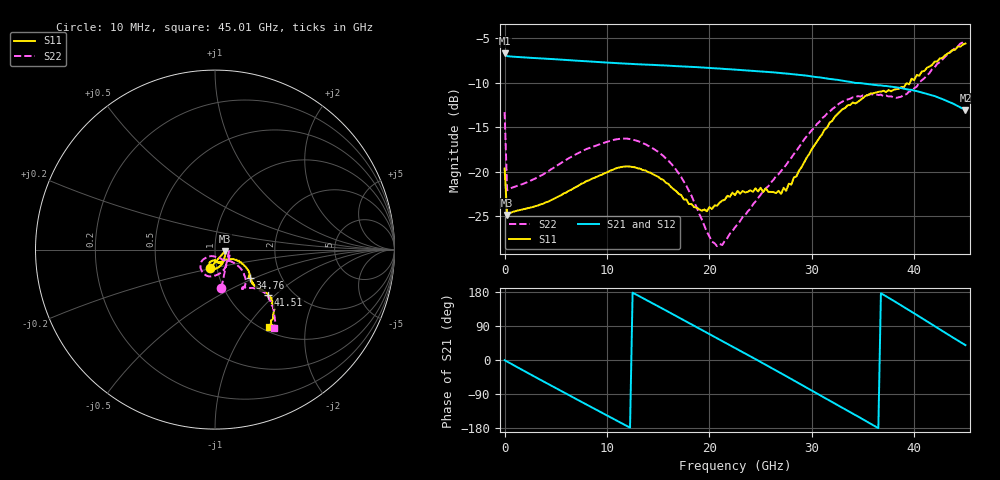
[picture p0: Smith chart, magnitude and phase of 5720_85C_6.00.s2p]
! Device:  ADRF5720
! Description: 0.5dB LSB GaAs MMIC 6-bit Digital Attenuator
! Frequency:  0.000009 -  40 GHz
! Ports:
!	RF1	= Port 1
!	RF2	= Port 2
! Vdd:  3.3 Volt
! Vss:  -3.3 Volt
! Control:  0/3.3 Volt
! State:  6.00 dB attenuation
! Data:  The device was measured using G-S-G Probes on a matrix board.
!  Data was collected using an calibrated 4 port network analyzer.
!  The reference plane for this measurement is at the launchers.
! Note:  Analog Devices supplies this data as a sample of measured data
!  for this product.  Your particular data for this product may vary.
!  Data was taken at 85 degrees C.
!  Analog Devices reserves the right to change this data at anytime.
# GHZ S DB R 45.0
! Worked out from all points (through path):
!   181 points, 10 MHz to 45.01 GHz, reference 45 ohm
!   highest |S21| = -6.71 dB at 10 MHz (marker M1); lowest = -13.1 dB at 45.01 GHz (marker M2)
!   group delay of S21, straight-line fit = 41.5 ps
!   lowest |S11| = -24.9 dB at 260 MHz (marker M3), VSWR 1.12, Z = 50.4 - j0.866 ohm
!   |S11| at or under -10 dB: start of sweep to 39.58 GHz
!   |S22| runs from -28.4 to -5.2 dB; largest |S21 - S12| = 0.0024
!   S11 on the Smith chart (normalised r, x): 10 MHz: 0.93, -0.19; 34.76 GHz: 1.39, -0.48; 41.51 GHz: 1.51, -0.91; 45.01 GHz: 1.07, -1.27
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0.01  -19.66 -104.2  -6.71 -0.4  -6.70 -0.4  -13.32 -80.5
0.26  -24.88 -8.6  -7.02 -4.0  -7.01 -4.0  -22.11 -6.9
2.01  -24.20 -16.4  -7.16 -30.3  -7.15 -30.2  -21.30 -19.7
4.26  -23.40 -38.1  -7.32 -63.2  -7.30 -63.2  -19.98 -45.4
6.01  -22.37 -49.9  -7.44 -88.7  -7.43 -88.6  -18.69 -61.0
7.76  -21.27 -60.7  -7.57 -114.0  -7.56 -113.9  -17.60 -74.6
11.51  -19.47 -87.8  -7.84 -167.9  -7.82 -167.8  -16.29 -103.6
13.26  -19.68 -99.6  -7.94 166.9  -7.92 167.1  -16.67 -116.4
15.26  -20.83 -109.8  -8.04 138.0  -8.03 138.2  -18.02 -130.2
17.76  -23.16 -108.4  -8.20 101.7  -8.18 101.9  -21.60 -139.9
20.26  -24.22 -86.6  -8.36 65.0  -8.34 65.2  -27.89 -116.9
21.26  -23.28 -80.5  -8.44 50.3  -8.42 50.5  -28.27 -91.7
22.76  -22.19 -74.0  -8.56 28.2  -8.54 28.4  -25.94 -66.0
24.76  -22.25 -70.4  -8.72 -1.4  -8.70 -1.2  -22.99 -52.3
27.01  -22.52 -51.9  -8.92 -35.1  -8.90 -34.8  -19.94 -38.5
30.26  -17.07 -27.1  -9.34 -84.5  -9.32 -84.2  -15.08 -36.1
32.26  -13.83 -30.2  -9.64 -114.9  -9.62 -114.6  -12.76 -43.0
34.76  -11.94 -39.2  -10.05 -152.8  -10.04 -152.5  -11.56 -53.4
37.76  -10.97 -41.9  -10.46 160.1  -10.44 160.5  -11.54 -54.6
39.76  -9.55 -41.6  -10.81 127.2  -10.80 127.6  -10.96 -49.1
41.51  -8.18 -40.6  -11.36 97.8  -11.33 98.2  -8.90 -41.1
45.01  -5.60 -55.3  -13.08 39.2  -13.05 39.6  -5.25 -52.9
